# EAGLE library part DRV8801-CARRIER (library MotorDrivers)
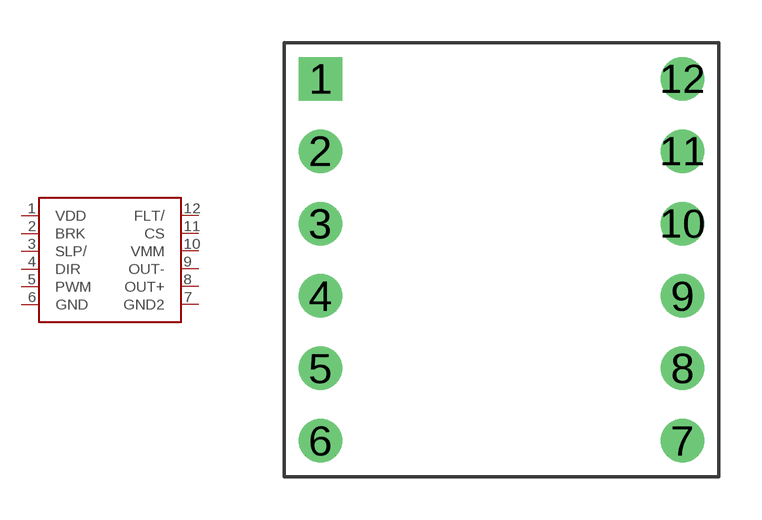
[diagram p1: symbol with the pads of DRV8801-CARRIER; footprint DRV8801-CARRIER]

Designator prefix -

## DRV8801-CARRIER  [DRV8801-CARRIER]
1  VDD
2  BRK
3  SLP/
4  DIR
5  PWM
6  GND
7  GND2
8  OUT+
9  OUT-
10  VMM
11  CS
12  FLT/

## Footprint DRV8801-CARRIER (pad centres in mm)
drill 1.016 square: 1 -6.35,6.35
drill 1.016: 2 -6.35,3.81; 3 -6.35,1.27; 4 -6.35,-1.27; 5 -6.35,-3.81; 6 -6.35,-6.35; 7 6.35,-6.35; 8 6.35,-3.81; 9 6.35,-1.27; 10 6.35,1.27; 11 6.35,3.81; 12 6.35,6.35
